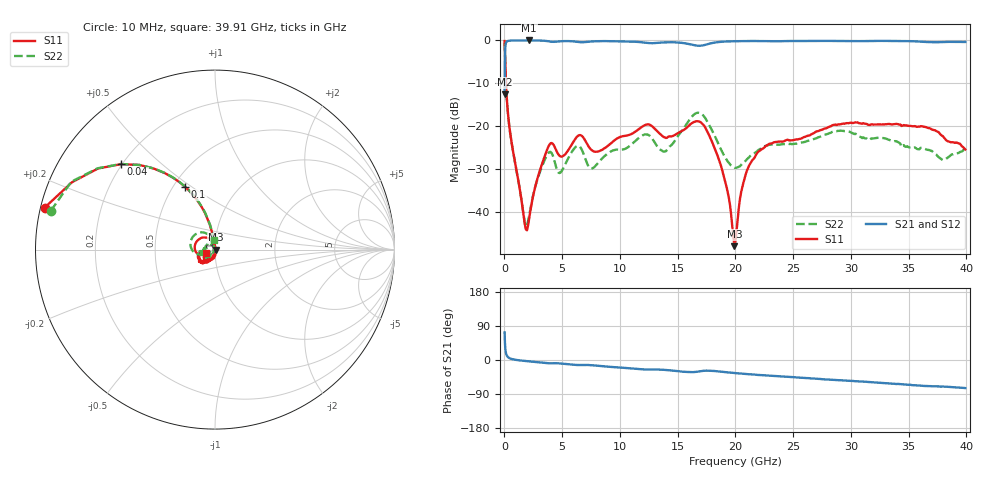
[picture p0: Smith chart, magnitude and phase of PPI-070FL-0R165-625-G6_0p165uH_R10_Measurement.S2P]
! Data measured by Modelithics Inc.  support@modelithics.com  813-866-6335  Tampa FL USA June 2025
! PPI-070FL-0R165-625-G6_0p165uH measured on 10-mil thick RO4350B board, mounted in 2-port shunt configuration on a 50-ohm transmission line
# Hz S MA R 50
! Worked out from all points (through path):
!   429 points, 10 MHz to 39.91 GHz, reference 50 ohm
!   highest |S21| = -0.05 dB at 2.145 GHz (marker M1); lowest = -12.5 dB at 10 MHz (marker M2)
!   group delay of S21, straight-line fit = 5.61 ps
!   lowest |S11| = -47.9 dB at 19.91 GHz (marker M3), VSWR 1.01, Z = 50.4 + j0.000818 ohm
!   |S11| at or under -10 dB: 127.2 MHz to end of sweep
!   |S22| runs from -43.4 to -0.5 dB; largest |S21 - S12| = 0.024
!   S11 on the Smith chart (normalised r, x): 10 MHz: 0.01, +0.12; 40 MHz: 0.20, +0.37; 100 MHz: 0.57, +0.47; 39.91 GHz: 0.90, -0.03
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1e7  0.9779 166.2  0.2359 73.1  0.2359 73.1  0.9396 166.7
4e7  0.7075 137.7  0.6731 45.0  0.6728 45.0  0.7096 137.8
1e8  0.3878 115.5  0.9035 22.6  0.9033 22.6  0.3885 115.4
2e8  0.2088 105.1  0.9665 11.7  0.9662 11.7  0.2092 104.8
4.941776e8  0.0829 99.8  0.9891 4.0  0.9889 4.0  0.08297 98.9
1.659243e9  0.009078 133.0  0.9936 -2.2  0.9933 -2.2  0.009244 134.0
2.144687e9  0.008571 -134.8  0.9938 -3.6  0.9935 -3.7  0.009293 -143.2
3.892285e9  0.06107 -122.4  0.9675 -8.8  0.9672 -8.8  0.0502 -141.1
4.766084e9  0.04532 -141.5  0.9718 -9.0  0.9716 -9.0  0.02855 -144.1
6.70786e9  0.07696 -144.3  0.947 -13.1  0.9466 -13.1  0.05291 -157.5
7.581659e9  0.05233 -145.5  0.9679 -13.9  0.9675 -13.9  0.03231 -141.9
1.214483e10  0.1028 -145.6  0.9376 -25.0  0.9372 -24.9  0.08012 -155.6
1.340699e10  0.08282 -167.5  0.9356 -25.1  0.9352 -25.2  0.05456 -174.7
1.729054e10  0.1013 140.4  0.8775 -28.4  0.8772 -28.3  0.1295 133.0
1.884396e10  0.03114 94.3  0.9608 -31.2  0.9605 -31.3  0.05051 109.1
1.991194e10  0.004029 0.1  0.9734 -34.2  0.9732 -34.4  0.03291 136.1
2.000902e10  0.004658 -36.2  0.9738 -34.5  0.9736 -34.6  0.0328 139.5
2.068865e10  0.02197 -80.8  0.9761 -36.1  0.9756 -36.3  0.03756 158.7
2.185371e10  0.04826 -98.0  0.9794 -39.3  0.979 -38.8  0.0509 171.5
2.670815e10  0.08211 -120.7  0.9821 -48.6  0.9817 -48.6  0.07043 -171.0
3.331019e10  0.1062 -137.6  0.9815 -61.8  0.9811 -62.0  0.06946 -168.1
3.991223e10  0.05365 -161.1  0.9549 -74.1  0.9544 -73.6  0.05611 94.7
